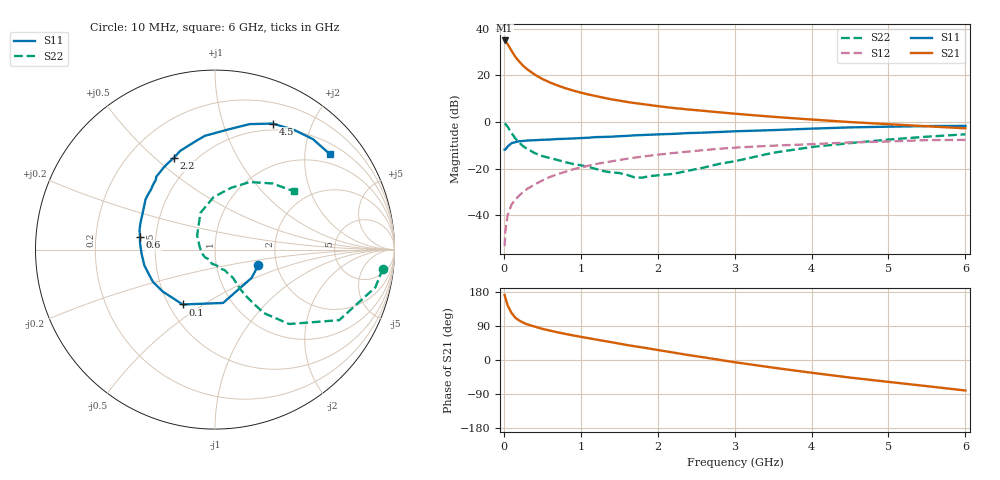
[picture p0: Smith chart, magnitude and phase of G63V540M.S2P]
! SIEMENS Small Signal Semiconductors
! BFG193
! Si NPN RF Bipolar Junction Transistor in SOT223
! VCE = 3.5 V  IC = 40 mA
! Common Emitter S-Parameters:  August  1996
# GHz  S  MA  R  50
!  f  S11  S21  S12  S22
! GHz  MAG  ANG  MAG  ANG  MAG  ANG  MAG  ANG
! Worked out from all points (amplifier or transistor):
!   36 points, 10 MHz to 6 GHz, reference 50 ohm
!   highest |S21| = 35.0 dB at 10 MHz (marker M1)
!   |S21| within 3 dB of that: start of sweep to 74.73 MHz
!   unconditionally stable (mu >= 1): 461.6 MHz to 2.402 GHz
!   at 250 MHz: K = 0.89, MSG = 27.1 dB, |S12| = -30.0 dB
!   at 1.4 GHz: K = 1.05, MAG = 12.0 dB, |S12| = -16.8 dB
!   at 6 GHz: K = 0.90, MSG = 2.5 dB, |S12| = -7.6 dB
!   S11 on the Smith chart (normalised r, x): 10 MHz: 1.60, -0.30; 100 MHz: 0.59, -0.41; 600 MHz: 0.41, +0.07; 2.2 GHz: 0.39, +0.58; 4.5 GHz: 0.42, +1.47; 6 GHz: 0.74, +2.57
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0.01  0.2566 -19.6  56.29 171.4  0.0022 86.6  0.9406 -6.5
0.02  0.2577 -37.7  54.46 164.2  0.0046 86.2  0.9181 -13.2
0.05  0.3008 -81.4  46.79 143.9  0.0104 71.6  0.7959 -29.6
0.1  0.3547 -120.5  33.83 124.1  0.0171 67.0  0.5853 -45.1
0.15  0.3731 -141.1  25.01 111.4  0.0221 64.8  0.4464 -52.4
0.2  0.3898 -152.5  19.85 104.2  0.0269 66.6  0.3647 -54.6
0.25  0.3953 -161.7  16.21 98.7  0.0316 66.8  0.3053 -56.4
0.3  0.4035 -167.6  13.74 94.4  0.0368 67.7  0.2701 -57.2
0.4  0.41 -177.0  10.48 88.2  0.0462 67.7  0.2177 -57.5
0.5  0.4189 175.3  8.422 82.2  0.0562 67.2  0.1879 -57.5
0.6  0.4237 170.6  7.082 77.6  0.067 66.6  0.1698 -58.7
0.7  0.4349 165.2  6.1 73.0  0.0768 65.2  0.1543 -61.1
0.8  0.4407 160.5  5.336 68.8  0.0865 63.3  0.1387 -63.0
1.1  0.4642 148.1  3.914 57.6  0.1165 58.2  0.1101 -74.5
1.3  0.4824 141.1  3.326 50.4  0.136 54.3  0.0891 -84.0
1.6  0.5081 130.7  2.711 39.6  0.1644 47.6  0.0743 -108.2
2.2  0.5604 114.1  2.014 19.8  0.2179 34.1  0.078 -172.1
2.8  0.6161 99.5  1.624 0.5  0.2689 20.2  0.1275 141.4
3.5  0.6754 83.3  1.301 -20.2  0.3135 3.0  0.2205 111.5
4.5  0.7723 65.4  1.004 -46.4  0.3676 -17.0  0.3553 75.5
5.5  0.8226 48.4  0.816 -69.0  0.4117 -40.2  0.4883 49.0
6  0.8317 39.9  0.738 -80.5  0.4176 -53.6  0.5482 36.2
